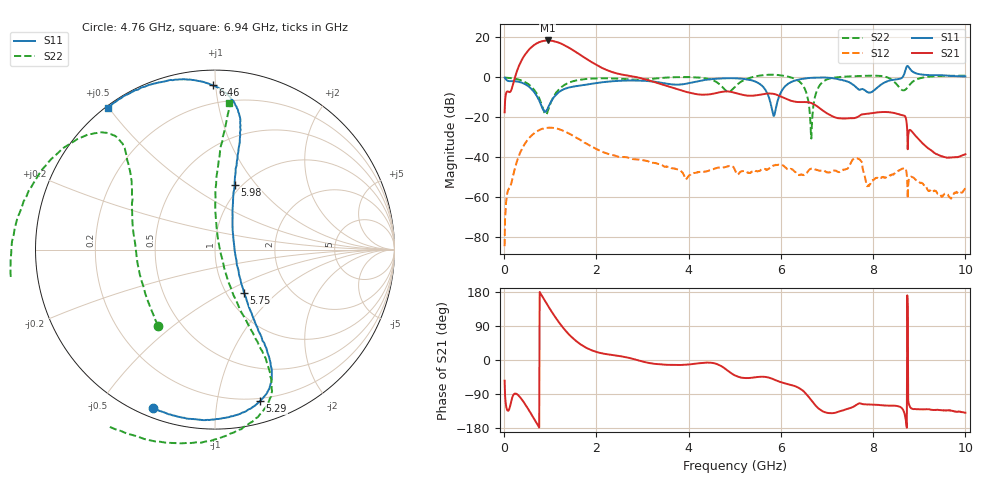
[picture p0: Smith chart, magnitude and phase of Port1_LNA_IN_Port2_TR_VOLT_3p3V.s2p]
! Created Tue Sep 16 14:21:07 2025
# hz S ma R 50
! 2 Port Network Data from SP1.SP block
! freq  magS11  angS11  magS21  angS21  magS12  angS12  magS22  angS22
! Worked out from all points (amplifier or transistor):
!   1000 points, 10 MHz to 10 GHz, reference 50 ohm
!   highest |S21| = 18.5 dB at 940 MHz (marker M1)
!   |S21| within 3 dB of that: 611.8 MHz to 1.359 GHz (747.3 MHz wide, 75.8 % of centre)
!   unconditionally stable (mu >= 1): start of sweep to 3.569 GHz; 4.193 GHz to 5.351 GHz; 6.219 GHz to 7.194 GHz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
!   at 1.67 GHz: K = 1.30, MAG = 18.0 dB, |S12| = -31.6 dB
!   at 5.01 GHz: K = 17.00, MAG = 4.2 dB, |S12| = -46.7 dB
!   at 10 GHz: K = 538.16, MSG = 8.4 dB, |S12| = -55.2 dB
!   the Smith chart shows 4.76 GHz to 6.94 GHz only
!   S11 on the Smith chart (normalised r, x): 4.76 GHz: 0.04, -0.68; 5.29 GHz: 0.18, -1.33; 5.75 GHz: 1.20, -0.64; 5.98 GHz: 0.93, +0.78; 6.46 GHz: 0.09, +0.98; 6.94 GHz: 0.01, +0.50
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1e7  0.986 -3.9  0.1334 -54.4  5.997e-05 -152.3  0.9939 -2.9
3.4e8  0.7635 -41.3  2.179 -97.6  0.0125 115.0  0.8633 -80.5
5.7e8  0.5424 -71.5  5.363 -139.1  0.03294 71.9  0.6134 -127.9
7.7e8  0.2465 -84.6  7.628 179.6  0.04872 32.9  0.2823 -159.2
9.4e8  0.1608 -24.2  8.38 145.0  0.05485 0.6  0.1358 -99.2
1.19e9  0.4295 -23.6  7.356 99.1  0.0507 -42.1  0.504 -100.4
1.41e9  0.5598 -52.7  5.481 66.9  0.03907 -71.6  0.7396 -123.3
1.68e9  0.6326 -89.1  3.476 39.4  0.02606 -96.9  0.8857 -135.7
2.12e9  0.7517 -123.3  1.727 17.7  0.01386 -115.6  0.9502 -132.6
3.34e9  0.7545 -111.2  0.713 -11.0  0.006846 -143.5  0.9497 -159.7
4.76e9  0.9463 -111.5  0.4416 -20.2  0.005571 -168.3  0.5286 -126.8
5.01e9  0.9497 -91.9  0.4072 -41.0  0.004602 158.9  0.5849 142.5
5.29e9  0.8809 -73.5  0.3488 -47.5  0.004048 172.6  0.9417 136.9
5.75e9  0.2914 -56.1  0.3958 -46.9  0.005359 169.4  1.166 -153.0
5.98e9  0.3766 73.1  0.3401 -57.7  0.006524 133.5  1.127 -112.3
6.46e9  0.915 90.8  0.2403 -79.2  0.003637 96.3  0.6698 -65.0
6.67e9  0.9775 104.7  0.2254 -108.1  0.005246 93.8  0.05958 73.4
6.94e9  0.9898 127.1  0.1393 -137.2  0.004606 81.3  0.818 84.4
7.72e9  0.4932 -152.8  0.1128 -114.4  0.008531 70.6  1.084 131.4
8.34e9  0.8235 122.2  0.1348 -120.4  0.00336 78.4  0.9665 -165.4
9.04e9  1.185 139.4  0.02453 -130.3  0.002303 79.0  0.9662 134.7
1e10  1.051 -167.6  0.01196 -139.0  0.001744 132.5  1.102 -167.7
